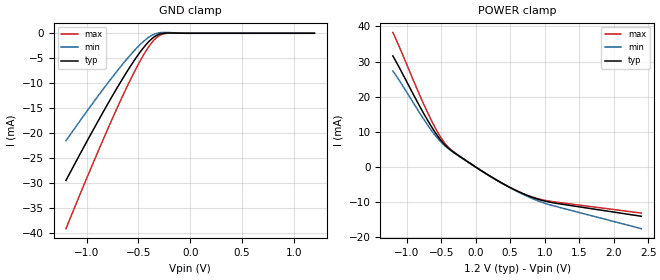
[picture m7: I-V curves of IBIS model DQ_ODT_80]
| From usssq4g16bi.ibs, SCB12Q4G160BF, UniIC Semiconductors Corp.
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|   Model DQ_ODT_80
[Model] DQ_ODT_80
Model_type Input
Polarity   Non-Inverting
Enable   Active-High
Vinl =  8.300E-01
Vinh =  9.700E-01
C_comp   8.151E-13   8.115E-13   8.151E-13
C_comp_power_clamp   2.538E-13   2.500E-13   2.636E-13
C_comp_gnd_clamp   5.577E-13   5.515E-13   5.651E-13
[Model Spec]
Vinh   9.700E-01   9.250E-01   1.015E+00
Vinl   8.300E-01   7.850E-01   8.750E-01
[Temperature Range]   45.000   95.000   -40.000
[Voltage Range]   1.200E+00   1.140E+00   1.260E+00
[C Comp Corner]
C_comp_power_clamp   2.538E-13   2.500E-13   2.636E-13
C_comp_gnd_clamp   5.577E-13   5.651E-13   5.515E-13
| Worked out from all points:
|   GND clamp passes 1 mA (typ) near -0.36 V on its own axis
|   POWER clamp passes 1 mA (typ) near -0.08 V on its own axis
[GND_clamp]
|Voltage   I(typ)   I(min)   I(max)
-1.2V     -29.48mA   -21.52mA   -39.13mA
-875mV    -17.04mA   -12.15mA   -22.94mA
-750mV    -12.49mA   -8.735mA   -17.01mA
-625mV    -8.165mA   -5.502mA   -11.35mA
-525mV    -4.976mA   -3.145mA   -7.147mA
-450mV    -2.86mA    -1.618mA   -4.313mA
-375mV    -1.172mA   -467.2uA   -1.971mA
-325mV    -429.2uA   -19.62uA   -862.4uA
-275mV    -56.59uA   156.6uA    -235.2uA
-200mV    56.62uA    142.6uA    17.87uA
-25mV     0A         0A         0A
1.2V      0A         0A         0A
[POWER_clamp]
|Voltage   I(typ)   I(min)   I(max)
-1.2V     31.62mA    27.33mA    38.31mA
-800mV    16.9mA     15.06mA    19.98mA
-625mV    11.02mA    9.999mA    12.65mA
-525mV    8.142mA    7.591mA    9.055mA
-450mV    6.389mA    6.12mA     6.847mA
-375mV    5.043mA    4.921mA    5.225mA
-300mV    3.948mA    3.875mA    4.044mA
350mV     -4.23mA    -4.224mA   -4.289mA
600mV     -6.809mA   -6.923mA   -6.823mA
825mV     -8.661mA   -9.014mA   -8.556mA
1.125V    -10.2mA    -11.03mA   -9.881mA
2.4V      -14.02mA   -17.54mA   -13.1mA
